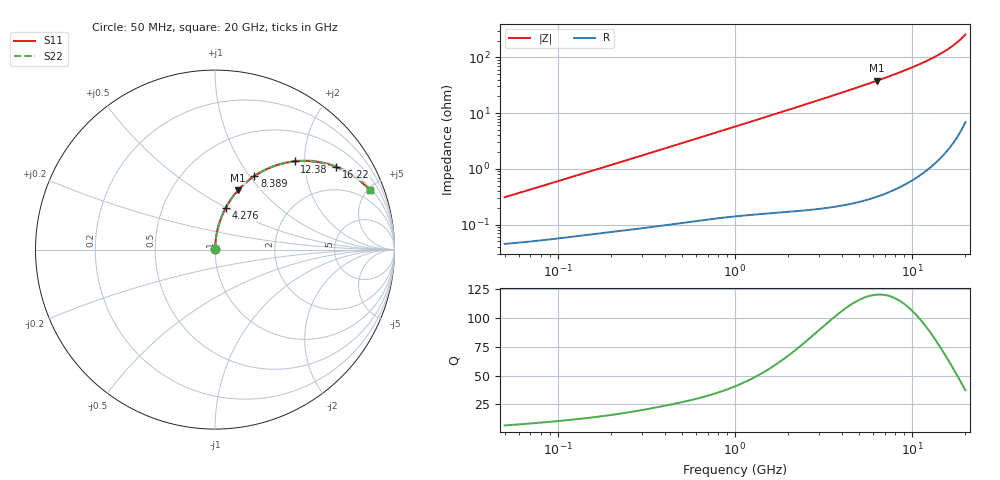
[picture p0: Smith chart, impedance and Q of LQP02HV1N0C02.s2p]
!Murata Part Number: LQP02HV1N0C02
!These Parameters are Measured in Series Mode Connection
!  o--[Z]--o
!Port1  Port2
!  o-------o
!Freq. Start=50[MHz] Stop=20[GHz], 401[Steps]
# Hz S RI R 50
!Freq.(Hz) S11(Real) S11(Imag) S21(Real) S21(Imag) S12(Real) S12(Imag) S22(Real) S22(Imag)
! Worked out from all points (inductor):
!   401 points, 50 MHz to 20 GHz, reference 50 ohm
!   read as one part in series: L = 968 pH near 51.52 MHz
!   highest Q = 120 at 6.312 GHz (marker M1), where L = 955 pH
!   S11 on the Smith chart (normalised r, x): 50 MHz: 1.00, +0.01; 4.276 GHz: 1.00, +0.50; 8.389 GHz: 1.01, +1.05; 12.38 GHz: 1.02, +1.79; 16.22 GHz: 1.05, +2.90; 20 GHz: 1.14, +5.13
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5e7  0.000461 0.00307  0.9995 -0.00307  0.9995 -0.00307  0.000461 0.00307
1.364002e8  0.000704 0.00809  0.9993 -0.00809  0.9993 -0.00809  0.000704 0.00809
3.721004e8  0.00141 0.0215  0.9986 -0.0215  0.9986 -0.0215  0.00141 0.0215
6.380365e8  0.00253 0.0366  0.9975 -0.0366  0.9975 -0.0366  0.00253 0.0366
1e9  0.00465 0.0569  0.9953 -0.0569  0.9953 -0.0569  0.00465 0.0569
1.714689e9  0.0111 0.0967  0.9889 -0.0967  0.9889 -0.0967  0.0111 0.0967
2.728004e9  0.0256 0.1522  0.9744 -0.1522  0.9744 -0.1522  0.0256 0.1522
3.415248e9  0.0391 0.1888  0.9609 -0.1888  0.9609 -0.1888  0.0391 0.1888
4.275624e9  0.0602 0.2333  0.9398 -0.2333  0.9398 -0.2333  0.0602 0.2333
5.273168e9  0.0902 0.2822  0.9098 -0.2822  0.9098 -0.2822  0.0902 0.2822
6.311513e9  0.1276 0.3295  0.8724 -0.3295  0.8724 -0.3295  0.1276 0.3295
7.442007e9  0.1749 0.3757  0.8251 -0.3757  0.8251 -0.3757  0.1749 0.3757
8.389408e9  0.2196 0.4096  0.7804 -0.4096  0.7804 -0.4096  0.2196 0.4096
9.316812e9  0.2671 0.438  0.7329 -0.438  0.7329 -0.438  0.2671 0.438
1.019291e10  0.3151 0.4598  0.6849 -0.4598  0.6849 -0.4598  0.3151 0.4598
1.131968e10  0.3802 0.4803  0.6198 -0.4803  0.6198 -0.4803  0.3802 0.4803
1.238412e10  0.4443 0.4913  0.5557 -0.4913  0.5557 -0.4913  0.4443 0.4913
1.438523e10  0.567 0.4889  0.433 -0.4889  0.433 -0.4889  0.567 0.4889
1.621653e10  0.6756 0.4601  0.3244 -0.4601  0.3244 -0.4601  0.6756 0.4601
1.774144e10  0.7585 0.4184  0.2415 -0.4184  0.2415 -0.4184  0.7585 0.4184
1.940974e10  0.8373 0.3571  0.1627 -0.3571  0.1627 -0.3571  0.8373 0.3571
2e10  0.8615 0.3322  0.1385 -0.3322  0.1385 -0.3322  0.8615 0.3322
